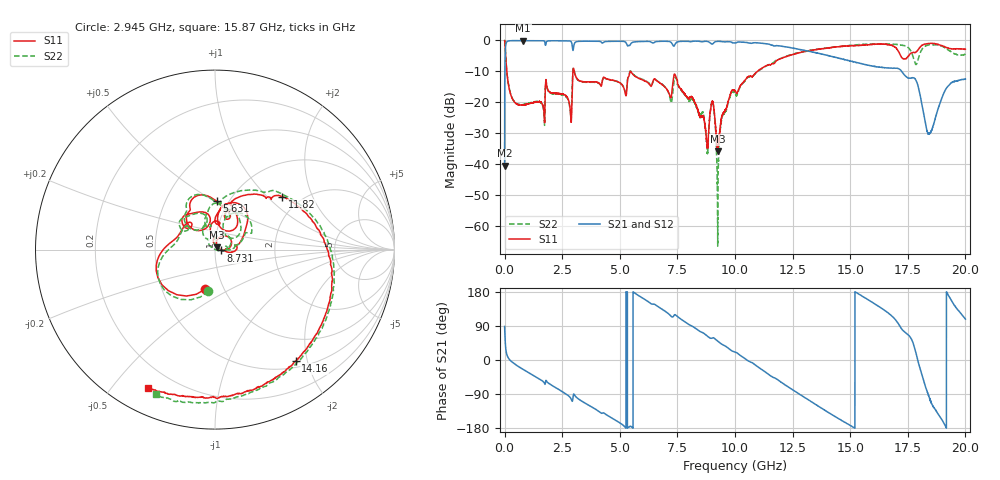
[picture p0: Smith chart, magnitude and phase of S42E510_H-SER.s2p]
!{S42E510}
!Johanson Technology Inc.
!www.johansontechnology.com
!Test Board Conditions:
!Substrate Type  RO4350B
!Substrate Thickness  50 mil
!Substrate Dk  3.66
!TL Type: GCPW
!TL Trace Width  60 mil
!TL Gap  10 mil
!Electrode orientation  Horizontal
!DUT TOPOLOGY	SERIES
!Mounting Pad LxW  14x55 mil
! Created Wed Nov 25 22:19:06 2020
# khz S ma R 50
! 2 Port Network Data from SP1.SP block
! freq  magS11  angS11  magS21  angS21  magS12  angS12  magS22  angS22
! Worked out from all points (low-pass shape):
!   20001 points, 300 kHz to 20 GHz, reference 50 ohm
!   highest |S21| = -0.05 dB at 806.3 MHz (marker M1); lowest = -40.4 dB at 300 kHz (marker M2)
!   |S21| within 3 dB of the highest: 31.27 MHz to 2.958 GHz (2.926 GHz wide, 196 % of centre); 2.978 GHz to 12.92 GHz (9.944 GHz wide, 125 % of centre)
!   lowest |S11| = -35.8 dB at 9.251 GHz (marker M3), VSWR 1.03, Z = 51 + j1.33 ohm
!   |S11| at or under -10 dB: 95.51 MHz to 2.965 GHz (2.869 GHz wide, 188 % of centre); 3.025 GHz to 5.458 GHz (2.433 GHz wide, 57.4 % of centre); 5.467 GHz to 10.97 GHz (5.501 GHz wide, 66.9 % of centre)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
!   |S22| runs from -66.4 to 0.0 dB; largest |S21 - S12| = 0.012
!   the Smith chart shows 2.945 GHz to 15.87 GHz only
!   S11 on the Smith chart (normalised r, x): 2.945 GHz: 0.81, -0.38; 5.631 GHz: 0.88, +0.51; 8.731 GHz: 1.07, -0.01; 11.82 GHz: 1.62, +1.24; 14.16 GHz: 0.60, -1.80; 15.87 GHz: 0.11, -0.62
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300  0.9963 -0.8  0.009596 88.5  0.009588 89.1  0.9961 -0.7
120300  0.2588 -79.7  0.9645 10.5  0.9655 10.5  0.2598 -79.5
806300  0.09083 -116.9  0.9948 -24.8  0.9932 -24.8  0.09203 -114.7
2945300  0.229 -104.5  0.7621 -108.3  0.7625 -108.3  0.2352 -99.1
3334300  0.2183 158.6  0.9703 -108.0  0.969 -108.0  0.2149 166.0
5631300  0.2697 88.1  0.9454 177.4  0.9449 177.4  0.2734 91.4
6667300  0.2151 54.4  0.964 140.5  0.9627 140.5  0.217 51.2
7421300  0.2681 48.0  0.8964 119.0  0.8968 119.0  0.2503 38.0
8731300  0.03377 -7.9  0.9685 66.5  0.969 66.5  0.03266 -4.8
9027300  0.1045 32.0  0.8776 58.6  0.8787 58.5  0.1057 39.4
9251300  0.01618 53.5  0.966 49.7  0.9675 49.7  0.001422 132.3
9462300  0.06437 96.2  0.9508 40.4  0.9493 40.4  0.06181 126.8
1.00003e7  0.1549 81.2  0.9088 20.9  0.9089 20.9  0.1419 100.5
1.18243e7  0.4781 38.2  0.824 -50.9  0.8236 -50.6  0.4847 39.9
1.33343e7  0.6937 -22.4  0.6513 -110.9  0.657 -110.8  0.697 -19.2
1.41603e7  0.7653 -54.1  0.5544 -142.6  0.562 -142.6  0.769 -50.2
1.58723e7  0.8565 -116.1  0.392 155.4  0.3919 155.1  0.8707 -112.5
1.66673e7  0.8535 -144.7  0.361 123.4  0.3527 124.1  0.8789 -142.8
1.78283e7  0.6406 -159.7  0.2386 25.1  0.2395 25.3  0.4211 -177.4
1.84243e7  0.8968 174.9  0.03122 -97.4  0.03128 -96.9  0.8476 -178.1
1.91833e7  0.7648 139.5  0.1714 179.4  0.1718 179.0  0.7315 144.0
2e7  0.7229 123.5  0.2373 108.0  0.24 108.9  0.5995 128.5
